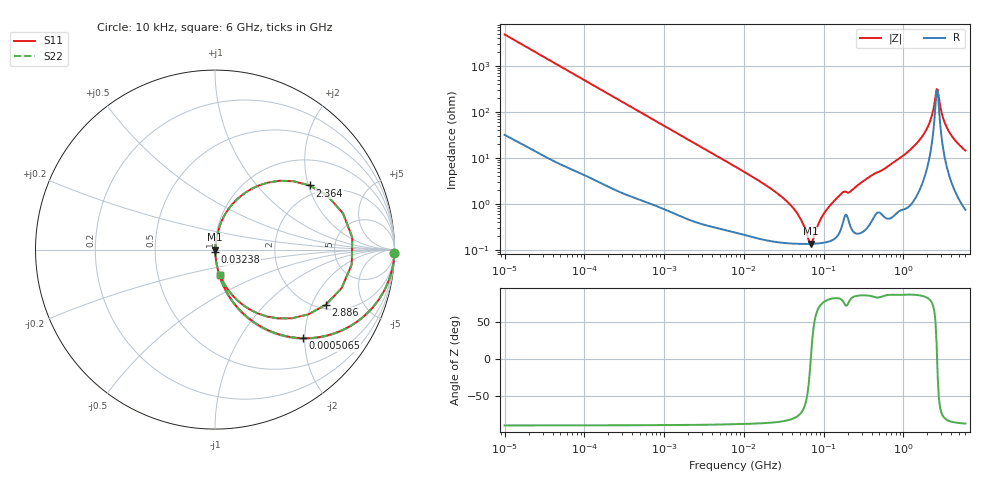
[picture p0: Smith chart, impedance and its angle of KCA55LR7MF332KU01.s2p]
!Murata Part Number: KCA55LR7MF332KU01
!These Parameters are Measured in Series Mode Connection
!Data Generated on Jan 08, 2026
!  o--ll--o
!Port1  Port2
!  o------o
!Operation Temp=25[degC], DC Bias Voltage=0[V]
!Freq. Start=10[kHz] Stop=6[GHz] 401[Steps]
# Hz S RI R 50
!Freq.(Hz) S11(Real) S11(Imag) S21(Real) S21(Imag) S12(Real) S12(Imag) S22(Real) S22(Imag)
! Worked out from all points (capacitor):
!   401 points, 10 kHz to 6 GHz, reference 50 ohm
!   read as one part in series: C = 3.26 nF near 10.69 kHz
!   lowest |Z| = 135 mohm at 69.58 MHz (marker M1)
!   series resonance near 69.06 MHz, so ESL is about 1.6 nH
!   S11 on the Smith chart (normalised r, x): 10 kHz: 2, -97; 506.5 kHz: 1.02, -1.96; 32.38 MHz: 1.00, -0.02; 2.364 GHz: 1.70, +2.04; 2.886 GHz: 2.17, -2.55; 6 GHz: 1.01, -0.29
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10000  0.9994 -0.0205  0.000555 0.0205  0.000555 0.0205  0.9994 -0.0205
92862  0.9641 -0.1818  0.0359 0.1818  0.0359 0.1818  0.9641 -0.1818
220506  0.8315 -0.3696  0.1685 0.3696  0.1685 0.3696  0.8315 -0.3696
506471  0.4899 -0.4938  0.5101 0.4938  0.5101 0.4938  0.4899 -0.4938
862344  0.2535 -0.4278  0.7465 0.4278  0.7465 0.4278  0.2535 -0.4278
1980684  0.064 -0.2359  0.936 0.2359  0.936 0.2359  0.064 -0.2359
7745967  0.00652 -0.0643  0.9935 0.0643  0.9935 0.0643  0.00652 -0.0643
3.237628e7  0.00155 -0.0124  0.9984 0.0124  0.9984 0.0124  0.00155 -0.0124
4.825823e7  0.00137 -0.00549  0.9986 0.00549  0.9986 0.00549  0.00137 -0.00549
6.957778e7  0.00134 0.000114  0.9987 -0.000114  0.9987 -0.000114  0.00134 0.000114
7.193098e7  0.00134 0.000616  0.9987 -0.000616  0.9987 -0.000616  0.00134 0.000616
9.70341e7  0.00143 0.00528  0.9986 -0.00528  0.9986 -0.00528  0.00143 0.00528
1.598104e8  0.00266 0.0151  0.9973 -0.0151  0.9973 -0.0151  0.00266 0.0151
6.67969e8  0.00935 0.0677  0.9907 -0.0677  0.9907 -0.0677  0.00935 0.0677
1.695223e9  0.0921 0.2475  0.9079 -0.2475  0.9079 -0.2475  0.0921 0.2475
2.069661e9  0.243 0.3568  0.757 -0.3568  0.757 -0.3568  0.243 0.3568
2.364181e9  0.5285 0.3571  0.4715 -0.3571  0.4715 -0.3571  0.5285 0.3571
2.612262e9  0.7649 0.0669  0.2351 -0.0669  0.2351 -0.0669  0.7649 0.0669
2.886376e9  0.6166 -0.3083  0.3834 0.3083  0.3834 0.3083  0.6166 -0.3083
3.189254e9  0.3517 -0.3834  0.6483 0.3834  0.6483 0.3834  0.3517 -0.3834
3.766309e9  0.1426 -0.2981  0.8574 0.2981  0.8574 0.2981  0.1426 -0.2981
6e9  0.0272 -0.139  0.9728 0.139  0.9728 0.139  0.0272 -0.139
